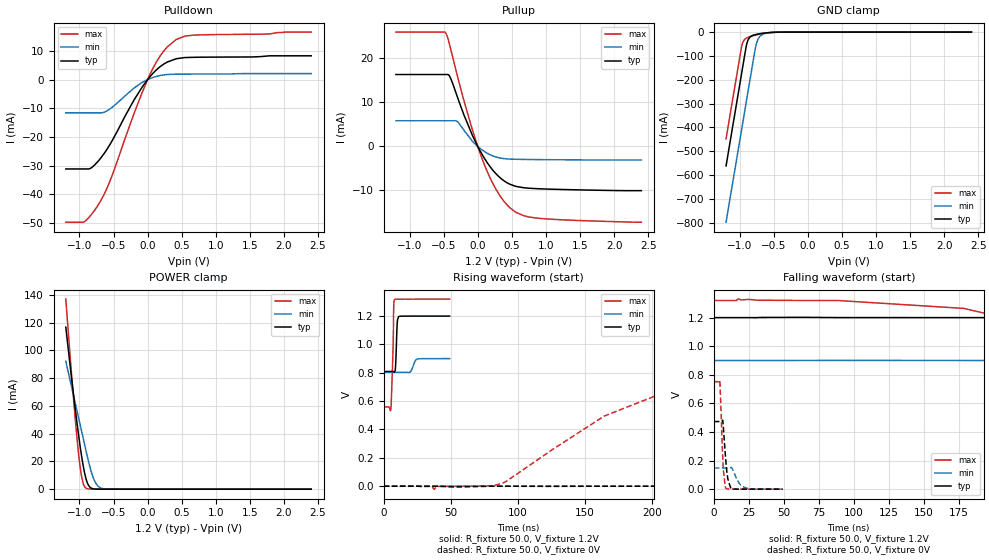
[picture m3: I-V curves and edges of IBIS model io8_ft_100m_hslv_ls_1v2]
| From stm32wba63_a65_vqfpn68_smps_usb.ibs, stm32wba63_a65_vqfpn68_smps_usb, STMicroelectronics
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[Model]   io8_ft_100m_hslv_ls_1v2
Model_type I/O
Polarity   Non-Inverting
Enable   Active-Low
| CAP_THRESHOLD on pad IOFT is "UDTCAPC" :
| Rising=30.0% of vddiom   Falling=70.0% of vddiom
| C_comp min and max val. don't necessarily correlate with the min and max pvt
| but are the smallest and greatest pad capacitance found.
| var   typ   min   max
C_comp   2.97447pF  2.89963pF  3.09649pF
|C_comp_pullup   1.72233pF  1.56276pF  1.88076pF
|C_comp_pulldown   1.25214pF  1.33687pF  1.21573pF
Vinl = 450.0mV
Vinh = 660.0mV
Vmeas = 600.0mV   | Reference voltage for timing measurements
Cref  = 50.0pF   | Timing specification test load capacitance value
Rref  = 1.0MOhm   | Timing specification test load resistance value
Vref  = 660.0mV   | Timing specification test load voltage
[Model Spec]
| TIME_THRESHOLD on pin ZIV11 is "CMOS" :
| Rising=50.0% of vdd   Falling=50.0% of vdd
Vinl 441.50000mV 335.50000mV 487.50000mV
Vinh 755.50000mV 552.50000mV 839.50000mV
| variable   typ   min   max
[Temperature Range] 25.0 140.0 -40.0
| variable   typ   min   max
[Voltage Range] 1.2V 900.0mV 1.32V
| variable   typ   min   max
[POWER Clamp Reference] 1.2V 900.0mV 1.32V
| variable   typ   min   max
[GND Clamp Reference] 0V 0V 0V
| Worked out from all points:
|   slope of the pulldown table from 0 to 0.18 V, typ, clamps not added: 40.6 ohm
|   slope of the pullup table from 0 to 0.18 V, typ, clamps not added: 39.4 ohm
|   GND clamp passes 1 mA (typ) near -0.51 V on its own axis
|   POWER clamp passes 1 mA (typ) near -0.83 V on its own axis
|   rising waveform, R_fixture 50.0, V_fixture 1.2V: 20-80 % time 863ps typ, 2.45ns min, 1.22ns max; typ from 0.809 V to 1.2 V
|   falling waveform, R_fixture 50.0, V_fixture 1.2V: 20-80 % time 322ns typ, 830ns min, 177ns max; typ from 1.2 V to 0.809 V
|   rising waveform, R_fixture 50.0, V_fixture 0V: 20-80 % time 368ns typ, 920ns min, 83.8ns max; typ from 0 V to 0.473 V
|   falling waveform, R_fixture 50.0, V_fixture 0V: 20-80 % time 2.49ns typ, 4.76ns min, 1.8ns max; typ from 0.473 V to 0 V
[POWER Clamp]
-1.2V     116.7mA    92.13mA    136.9mA
-1.09V    69.42mA    68.21mA    67.14mA
-1.02V    41.75mA    52.99mA    28.91mA
-990mV    30.98mA    46.47mA    16.09mA
-970mV    24.36mA    42.12mA    9.575mA
-940mV    15.59mA    35.6mA     3.485mA
-910mV    8.693mA    29.07mA    1.01mA
-860mV    2.259mA    18.59mA    104.6uA
-780mV    143.1uA    6.246mA    2.554uA
-720mV    16.22uA    1.846mA    157.1nA
-650mV    1.267uA    330.3uA    6.114nA
2.4V      0A         0A         0A
[GND Clamp]
-1.2V     -561.6mA   -797.4mA   -447.4mA
-980mV    -187.6mA   -423.4mA   -73.43mA
-960mV    -153.6mA   -389.4mA   -48.26mA
-900mV    -54.17mA   -287.4mA   -24.97mA
-870mV    -29.55mA   -236.4mA   -21.19mA
-830mV    -17.05mA   -168.4mA   -17.42mA
-760mV    -9.921mA   -54.55mA   -11.89mA
-730mV    -8.191mA   -29.78mA   -9.811mA
-690mV    -6.26mA    -14.49mA   -7.318mA
-600mV    -2.976mA   -4.315mA   -3.058mA
-380mV    -57.63uA   -251uA     -19.49uA
2.4V      871.4pA    205.6nA    347.3pA
| variable   typ   min   max
[Pullup Reference] 1.2V 900.0mV 1.32V
| variable   typ   min   max
[Pulldown Reference] 0V 0V 0V
[Pullup]
-1.2V     16.33mA    5.833mA    25.98mA
-470mV    16.33mA    5.833mA    25.81mA
-410mV    15.87mA    5.833mA    22.96mA
-300mV    11.32mA    5.662mA    16.14mA
-80mV     2.58mA     1.232mA    3.849mA
80mV      -2.237mA   -962.5uA   -3.434mA
190mV     -4.777mA   -1.94mA    -7.418mA
310mV     -6.857mA   -2.571mA   -10.82mA
540mV     -8.979mA   -2.909mA   -14.76mA
670mV     -9.371mA   -2.948mA   -15.71mA
920mV     -9.627mA   -2.991mA   -16.35mA
2.4V      -10.04mA   -3.074mA   -17.21mA
[Pulldown]
-1.2V     -31.2mA    -11.62mA   -49.78mA
-930mV    -31.2mA    -11.62mA   -49.64mA
-830mV    -30.86mA   -11.62mA   -47.25mA
-710mV    -28.04mA   -11.62mA   -43.19mA
-550mV    -22.55mA   -10.2mA    -35.3mA
-200mV    -7.146mA   -2.964mA   -11.89mA
40mV      1.171mA    405.7uA    2.092mA
130mV     3.416mA    1.118mA    6.182mA
230mV     5.302mA    1.612mA    9.763mA
420mV     7.288mA    1.898mA    13.99mA
670mV     7.779mA    1.924mA    15.51mA
2.4V      8.3mA      2.094mA    16.59mA
[Ramp]
dV/dt_r 283.78522mV/72.68388ns 88.90596mV/182.66143ns 450.99479mV/15.99476ns
dV/dt_f 234.65959mV/62.80682ns 57.87864mV/163.97055ns 456.7356mV/34.0031ns
R_load = 50.0
| Removed startup time: 0s 0s 0s  .
| Removed end time: 49.2ns.
[Rising Waveform]
R_fixture   = 50.0
V_fixture   = 1.2V
V_fixture_min = 900.0mV
V_fixture_max = 1.32V
0s        808.9mV    803.5mV    558.8mV
5.45ns    808.9mV    803.5mV    553.4mV
7.1ns     808.8mV    803.5mV    998.1mV
7.5ns     807.6mV    803.5mV    1.264V
8.05ns    804.4mV    803.5mV    1.316V
8.95ns    859.2mV    803.5mV    1.319V
10.2ns    1.161V     803.5mV    1.319V
11.05ns   1.195V     803.5mV    1.319V
25.15ns   1.2V       897.3mV    1.32V
49.2ns    1.2V       899.9mV    1.32V
| Removed startup time: 0s 0s 0s  .
| Removed end time: 9.99625us.
[Falling Waveform]
R_fixture   = 50.0
V_fixture   = 1.2V
V_fixture_min = 900.0mV
V_fixture_max = 1.32V
0s        1.2V       900mV      1.32V
178.5ns   1.2V       900.2mV    1.264V
325.5ns   1.196V     900mV      815.7mV
408ns     1.17V      900mV      688.2mV
495.3ns   1.104V     900mV      625.6mV
738ns     907.2mV    899.7mV    571.7mV
1.02us    838.6mV    896.2mV    560.9mV
1.632us   811.6mV    847.7mV    558.8mV
3.264us   808.9mV    806.4mV    558.8mV
9.996us   808.9mV    803.5mV    558.8mV
| Removed startup time: 0s 0s 0s  .
| Removed end time: 9.99625us.
[Rising Waveform]
R_fixture   = 50.0
V_fixture   = 0V
V_fixture_min = 0V
V_fixture_max = 0V
0s        4.602nV    216.1nV    3.171nV
87ns      -111.6uV   55.8uV     16.49mV
164.3ns   -99.15uV   -27.42uV   493.9mV
204ns     33.29uV    -26.17uV   642.2mV
408ns     88.06mV    -5.968uV   750.3mV
612ns     278.4mV    209.4uV    751.5mV
816ns     393.4mV    1.347mV    751.6mV
1.278us   463.9mV    35.98mV    751.6mV
2.856us   472.8mV    140.7mV    751.6mV
9.996us   473mV      148.2mV    751.7mV
| Removed startup time: 0s 0s 0s  .
| Removed end time: 49.2ns.
[Falling Waveform]
R_fixture   = 50.0
V_fixture   = 0V
V_fixture_min = 0V
V_fixture_max = 0V
0s        473mV      148.3mV    751.7mV
4.3ns     473mV      148.3mV    756.3mV
6.3ns     482.5mV    148.3mV    242.4mV
6.65ns    455.6mV    148.3mV    169.9mV
8.5ns     209.7mV    148.3mV    8.426mV
10.05ns   72.28mV    148.2mV    1.76mV
12.5ns    4.124mV    152.5mV    486uV
18.1ns    276uV      41.82mV    171.9uV
21.1ns    127.2uV    16.01mV    157.6uV
49.2ns    84.9uV     25.03uV    177.9uV
